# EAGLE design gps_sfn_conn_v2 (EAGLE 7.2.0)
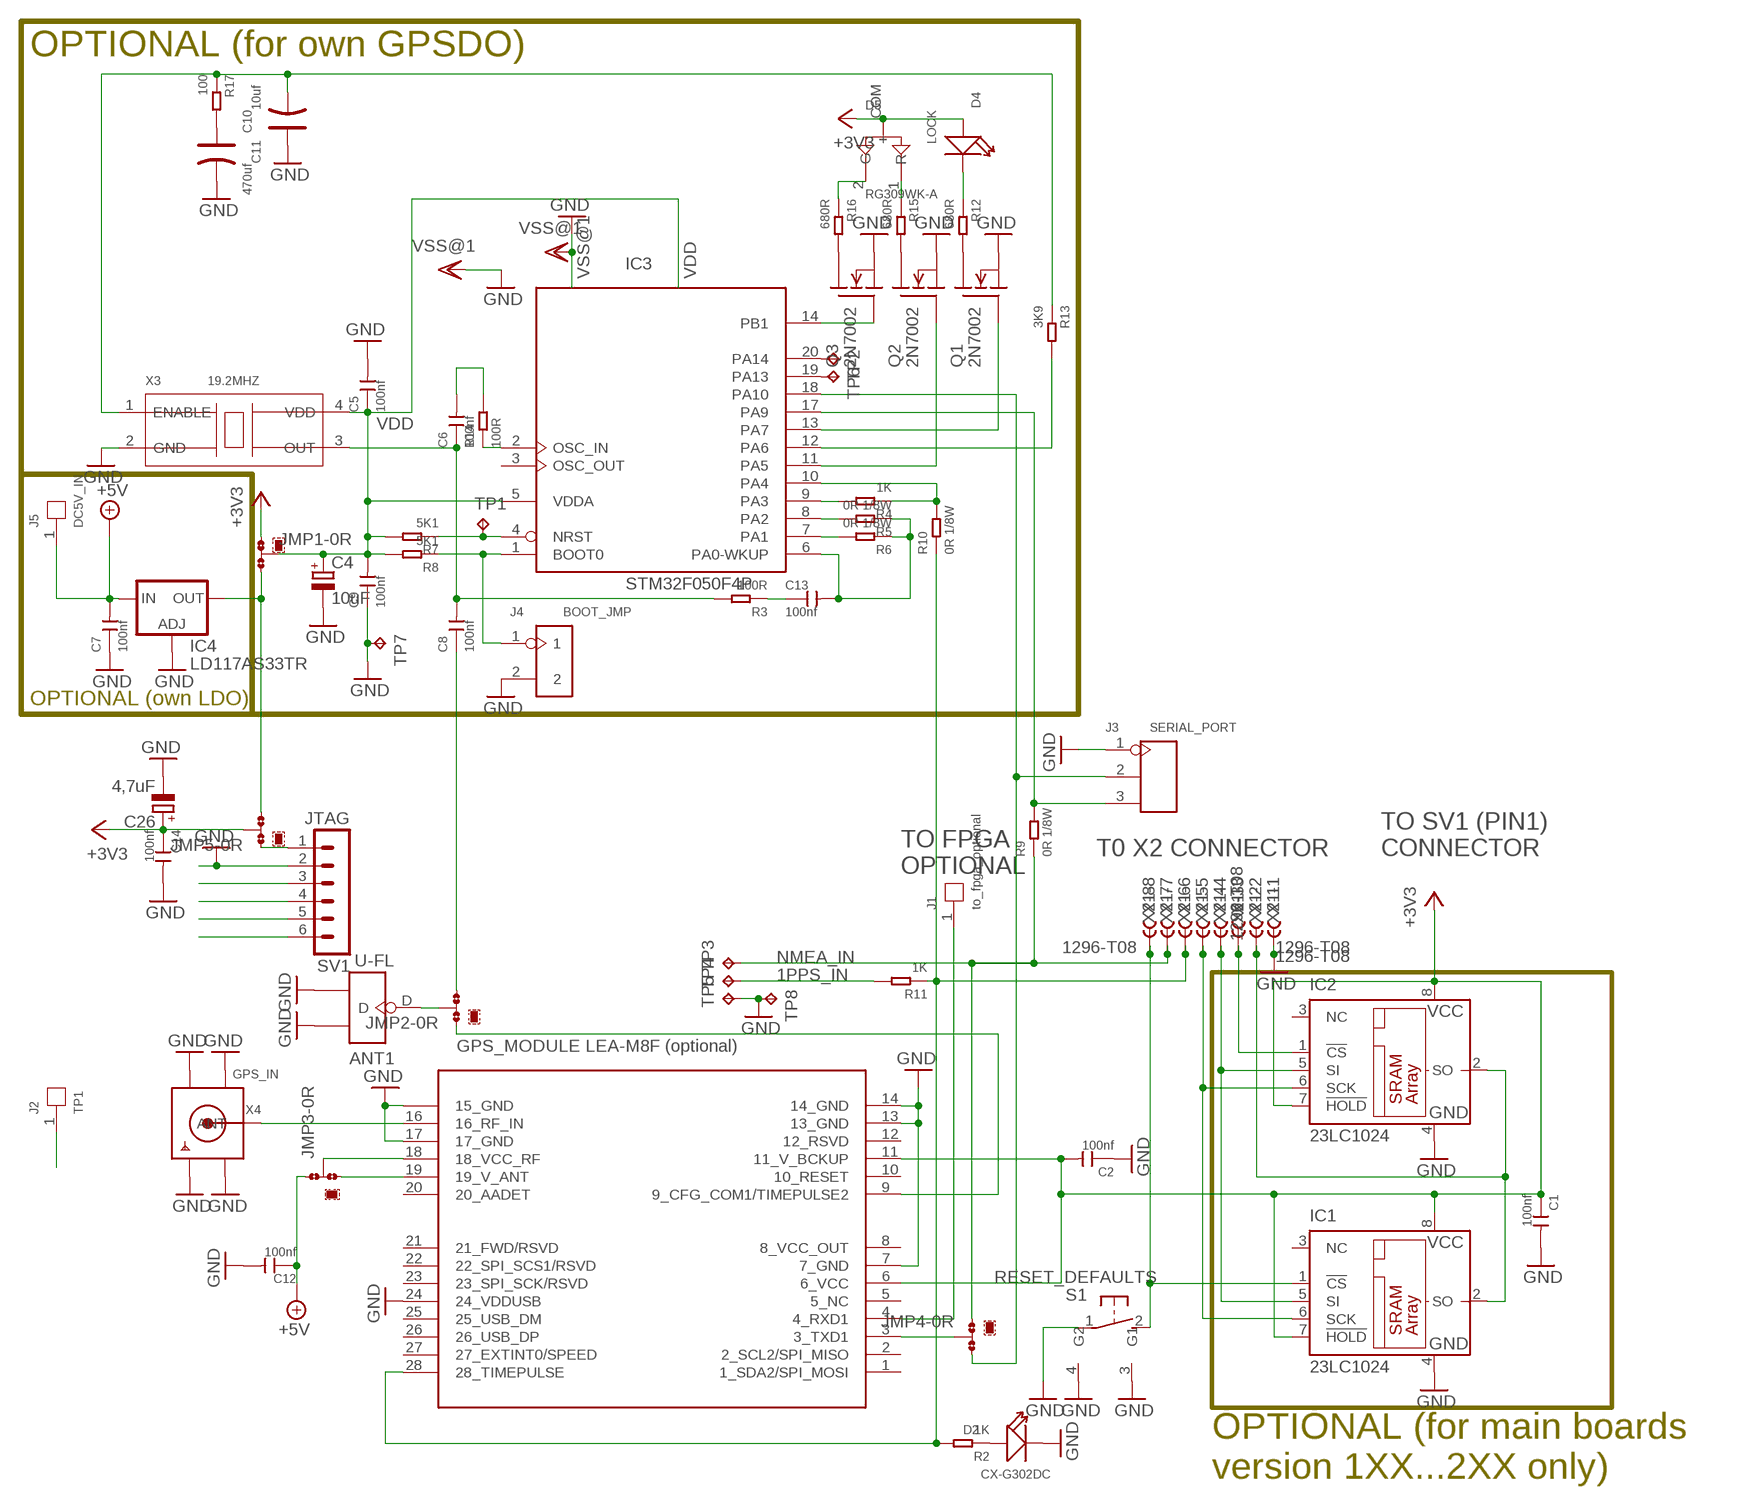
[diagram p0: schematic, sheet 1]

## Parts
ANT1  U-FL  ANTENNA-CONN-U-FL(3P)  [U-FL3P-SMD-2.6X2.6X1.0MM]
C1  100nf  CERAMIC-100NF-50V-10%-X7R(0805)  [C0805]
C2  100nf  CERAMIC-100NF-50V-10%-X7R(0805)  [C0805]
C4  10uF  CPOL-EUA/3216-18R  [A/3216-18R]
C5  100nf  CERAMIC-100NF-50V-10%-X7R(0805)  [C0805]
C6  100nf  CERAMIC-100NF-50V-10%-X7R(0805)  [C0805]
C7  100nf  CERAMIC-100NF-50V-10%-X7R(0805)  [C0805]
C8  100nf  CERAMIC-100NF-50V-10%-X7R(0805)  [C0805]
C9  100nf  CERAMIC-100NF-50V-10%-X7R(0805)  [C0805]
C10  470uf  TANTALUM-SMD-470UF-6.3V(AVX-D)  [AVX-D]
C11  10uf  TANTALUM-SMD-10UF-10V-10%(AVX-A)  [AVX-A]
C12  100nf  CERAMIC-100NF-50V-10%-X7R(0805)  [C0805]
C13  100nf  CERAMIC-100NF-50V-10%-X7R(0805)  [C0805]
C14  100nf  CERAMIC-100NF-50V-10%-X7R(0805)  [C0805]
C26  4,7uF  CPOL-EUA/3216-18R  [A/3216-18R]
D2  CX-G302DC  DIP-LED-GREEN-GREEN(2P-D3MM)  [LED2-2.54-D3.0MM]
D4  LOCK  DIP-LED-GREEN-GREEN(2P-D3MM)  [LED2-2.54-D3.0MM]
D5  RG309WK-A  DIP-LED-RED/GREEN-COMMON-CATHODE(3P-2.54)  [LED3-2.54-D3.0MM]
IC1  23LC1024  23SOIC  [SO-08]
IC2  23LC1024  23SOIC  [SO-08]
IC3  STM32F050F4P  [TSSOP20-I]
IC4  LD117AS33TR  [SOT223]
J1  to_fpga_optional  DIP-BLACK-ROUND-FEMALE-HEADER-VERT(1P-2.54)  [1P-65/35MIL]
J2  TP1  DIP-BLACK-ROUND-FEMALE-HEADER-VERT(1P-2.54)  [1P-65/35MIL]
J3  SERIAL_PORT  DIP-BLACK-FEMALE-HEADER-VERT(3P-2.54)  [H3-2.54]
J4  BOOT_JMP  DIP-BLACK-FEMALE-HEADER-VERT(2P-2.54)  [H2-2.54]
J5  DC5V_IN  DIP-BLACK-ROUND-FEMALE-HEADER-VERT(1P-2.54)  [1P-65/35MIL]
JMP1  0R-JUMPA  [A0R-JMP]
JMP2  0R-JUMPA  [A0R-JMP]
JMP3  0R-JUMPA  [A0R-JMP]
JMP4  0R-JUMPA  [A0R-JMP]
JMP5  0R-JUMPA  [A0R-JMP]
Q1  2N7002  [SOT23]
Q2  2N7002  [SOT23]
Q3  2N7002  [SOT23]
R2  1K  SMD-RES-0R-5%-1/8W(0805)  [R0805]
R3  100R  SMD-RES-0R-5%-1/8W(0805)  [R0805]
R4  1K  SMD-RES-0R-5%-1/8W(0805)  [R0805]
R5  0R 1/8W  SMD-RES-0R-5%-1/8W(0805)  [R0805]
R6  0R 1/8W  SMD-RES-0R-5%-1/8W(0805)  [R0805]
R7  5K1  SMD-RES-0R-5%-1/8W(0805)  [R0805]
R8  5K1  SMD-RES-0R-5%-1/8W(0805)  [R0805]
R9  0R 1/8W  SMD-RES-0R-5%-1/8W(0805)  [R0805]
R10  0R 1/8W  SMD-RES-0R-5%-1/8W(0805)  [R0805]
R11  1K  SMD-RES-0R-5%-1/8W(0805)  [R0805]
R12  680R  SMD-RES-0R-5%-1/8W(0805)  [R0805]
R13  3K9  SMD-RES-0R-5%-1/8W(0805)  [R0805]
R14  100R  SMD-RES-0R-5%-1/8W(0805)  [R0805]
R15  680R  SMD-RES-0R-5%-1/8W(0805)  [R0805]
R16  680R  SMD-RES-0R-5%-1/8W(0805)  [R0805]
R17  100  SMD-RES-0R-5%-1/8W(0805)  [R0805]
S1  RESET_DEFAULTS  31-XX  [B3F-31XX]
SV1  JTAG  MA06-1  [MA06-1]
TP1  UART_OUT  TPB1,27  [B1,27]
TP2  UART_OUT  TPB1,27  [B1,27]
TP3  UART_OUT  TPB1,27  [B1,27]
TP4  UART_OUT  TPB1,27  [B1,27]
TP5  UART_OUT  TPB1,27  [B1,27]
TP6  UART_OUT  TPB1,27  [B1,27]
TP7  UART_OUT  TPB1,27  [B1,27]
TP8  UART_OUT  TPB1,27  [B1,27]
UBLOX_LEA-M8F  UBLOX_LEA-M8F/Quectel L10  UBLOX_LEA-6  [UBLOX_LEA-6T]
X1  1296-T08  [1296-08]
X2  1296-T08  [1296-08]
X3  19.2MHZ  SMD-CRYSTAL-16MHZ-9PF-10PPM-60R(4P-3.2X2.5MM)  [X4-SMD-3.2X2.5X0.7MM]
X4  GPS_IN  SMACONNECTOR_EDGE_UFL  [SMA_EDGELAUNCH_UFL]

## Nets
1PPS_IN: R2.2 R10.1 R11.1 UBLOX_LEA-M8F.28(28_TIMEPULSE) X1.6 X2.6
+3V3: C1.1 C2.2 C14.1 C26.+ D4.A(+) D5.COM(+) IC1.7(!HOLD) IC1.8(VCC) IC2.7(!HOLD) IC2.8(VCC) JMP1.1 JMP5.2 UBLOX_LEA-M8F.6(6_VCC) UBLOX_LEA-M8F.11(11_V_BCKUP)
+5V: C7.2 C12.1 IC4.3(IN) J5.1 JMP3.1
GND: ANT1.GND1 ANT1.GND2 C1.2 C2.1 C4.- C5.2 C7.1 C9.1 C10.- C11.+ C12.2 C14.2 C26.- D2.K(-) IC1.4(GND) IC2.4(GND) IC4.1(ADJ) J3.1 J4.2 Q1.2(S) Q2.2(S) Q3.2(S) S1.1(P) S1.3(G1) S1.4(G2) SV1.2 TP5.TP TP7.TP TP8.TP UBLOX_LEA-M8F.7(7_GND) UBLOX_LEA-M8F.13(13_GND) UBLOX_LEA-M8F.14(14_GND) UBLOX_LEA-M8F.15(15_GND) UBLOX_LEA-M8F.17(17_GND) UBLOX_LEA-M8F.24(24_VDDUSB) X1.1 X2.1 X3.2(GND) X4.GND@1(GND1) X4.GND@2(GND2) X4.GND@3(GND3) X4.GND@4(GND4)
N$1: SV1.6
N$2: SV1.5
N$3: SV1.4
N$4: SV1.3
N$5: IC1.1(!CS) S1.2(S) X1.8 X2.8
N$6: JMP3.3 UBLOX_LEA-M8F.19(19_V_ANT)
N$7: IC1.2(SO) IC2.2(SO) X1.2 X2.2
N$8: IC2.1(!CS) X1.3 X2.3
N$9: IC1.5(SI) IC2.5(SI) X1.4 X2.4
N$10: IC1.6(SCK) IC2.6(SCK) X1.5 X2.5
N$11: J1.1 UBLOX_LEA-M8F.4(4_RXD1)
N$12: D2.A(+) R2.1
N$13: UBLOX_LEA-M8F.16(16_RF_IN) X4.P(ANT)
N$14: JMP3.2 UBLOX_LEA-M8F.18(18_VCC_RF)
N$15: JMP2.1 UBLOX_LEA-M8F.9(9_CFG_COM1/TIMEPULSE2)
N$16: R11.2 TP4.TP
N$17: IC3.20(PA14) TP2.TP
N$18: ANT1.D JMP2.2
N$19: J2.1
N$20: IC3.4(NRST) R7.1 TP1.TP
N$21: IC3.1(BOOT0) J4.1 R8.1
N$22: C13.2 IC3.6(PA0-WKUP) R5.1 R6.1
N$23: JMP4.2 UBLOX_LEA-M8F.3(3_TXD1)
N$24: C13.1 R3.1
N$25: C6.1 C8.2 R3.2 X3.3(OUT)
N$26: IC3.9(PA3) R4.2
N$27: IC3.10(PA4) R4.1 R10.2
N$28: IC3.7(PA1) R6.2
N$29: IC3.2(OSC_IN) R14.1
N$30: IC3.8(PA2) R5.2
N$31: IC4.4(OUT) JMP1.3 JMP5.3
N$32: C6.2 R14.2
N$33: JMP5.1 SV1.1
N$34: C8.1 JMP2.3
N$35: IC3.18(PA10) J3.2 JMP4.3
N$36: IC3.17(PA9) J3.3 R9.2
N$37: IC3.12(PA6) R13.2
N$38: C10.+ R17.2
N$39: C11.- R13.1 R17.1 X3.1(ENABLE)
N$40: D5.1(R) R15.1
N$41: D5.2(G) R16.1
N$42: D4.K(-) R12.1
N$43: IC3.14(PB1) Q3.1(G)
N$44: IC3.11(PA5) Q2.1(G)
N$45: IC3.13(PA7) Q1.1(G)
N$46: IC3.19(PA13) TP6.TP
N$47: Q1.3(D) R12.2
N$48: Q2.3(D) R15.2
N$49: Q3.3(D) R16.2
NMEA_IN: JMP4.1 R9.1 TP3.TP X1.7 X2.7
VDD: C4.+ C5.1 C9.2 IC3.5(VDDA) JMP1.2 R7.2 R8.2 X3.4(VDD)
Unconnected: IC1.3(NC) IC2.3(NC) IC3.3(OSC_OUT) UBLOX_LEA-M8F.1(1_SDA2/SPI_MOSI) UBLOX_LEA-M8F.2(2_SCL2/SPI_MISO) UBLOX_LEA-M8F.5(5_NC) UBLOX_LEA-M8F.8(8_VCC_OUT) UBLOX_LEA-M8F.10(10_RESET) UBLOX_LEA-M8F.12(12_RSVD) UBLOX_LEA-M8F.20(20_AADET) UBLOX_LEA-M8F.21(21_FWD/RSVD) UBLOX_LEA-M8F.22(22_SPI_SCS1/RSVD) UBLOX_LEA-M8F.23(23_SPI_SCK/RSVD) UBLOX_LEA-M8F.25(25_USB_DM) UBLOX_LEA-M8F.26(26_USB_DP) UBLOX_LEA-M8F.27(27_EXTINT0/SPEED)

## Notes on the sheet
- OPTIONAL (for own GPSDO)
- OPTIONAL (own LDO)
- T0 X2 CONNECTOR
- TO SV1 (PIN1)
  CONNECTOR
- TO FPGA
  OPTIONAL
- GPS_MODULE LEA-M8F (optional)
- OPTIONAL (for main boards
  version 1XX...2XX only)

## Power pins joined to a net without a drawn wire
VDD: IC3.16(VDD)
VSS@1: IC3.15(VSS)

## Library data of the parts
ANT1 = Seeed-OPL-Connector:ANTENNA-CONN-U-FL(3P): 320110048
C1 C2 C5-C9 C12-C14 = Seeed-OPL-Capacitor:CERAMIC-100NF-50V-10%-X7R(0805): 302010165; MPN: CC0805KRX7R9BB104
C4 C26 = rcl:CPOL-EU: POLARIZED CAPACITOR, European symbol
C10 = Seeed-OPL-Capacitor:TANTALUM-SMD-470UF-6.3V(AVX-D): 302020027
C11 = Seeed-OPL-Capacitor:TANTALUM-SMD-10UF-10V-10%(AVX-A): 302020011; MPN: TAJA106K010RNJ
D2 = Seeed-OPL-Diode:DIP-LED-GREEN-GREEN(2P-D3MM): 304090040; MPN: CX-G302DC
D4 = Seeed-OPL-Diode:DIP-LED-GREEN-GREEN(2P-D3MM): 304090040; MPN: CX-G302DC; VALUE: CX-G302DC
D5 = Seeed-OPL-Diode:DIP-LED-RED/GREEN-COMMON-CATHODE(3P-2.54): 304090022; MPN: RG309WK-A
IC1 IC2 = W5500_LX9_AD9957:23*: Serial EEPROM 4K/ 8K , SPI bus
IC3 = micro-stm_v3:STM32F050F*P: ARM 32-bit Cortex™-M0 CPU 48 MHz maximum frequency 16to 32 Kbytes of Flash memory 4 kbytes of SRAM 15 GPIOs 2.0 to 3.6 V application supply
IC4 = W5500_LX9_AD9957:LD117A?*: Low drop fixed and adjustable positive voltage regulators 1 A Source: http://www.st.com/stonline/products/literature/ds/7194/ld1117axx.pdf
J1 J2 J5 = Seeed-OPL-Connector:DIP-BLACK-ROUND-FEMALE-HEADER-VERT(1P-2.54): 320030026; MPN: RF130-1013BBS0741; VALUE: 1p-2.54
J3 = Seeed-OPL-Connector:DIP-BLACK-FEMALE-HEADER-VERT(3P-2.54): 320030024; MPN: F185-1103A0BSYA1; VALUE: 3p-2.54
J4 = Seeed-OPL-Connector:DIP-BLACK-FEMALE-HEADER-VERT(2P-2.54): 320030023; MPN: F185-1102A1BSYA1; VALUE: 2p-2.54
JMP1-JMP5 = W5500_LX9_AD9957:0R-JUMP: SMD 0R 0805 Jumper
Q1-Q3 = transistors_gaui:2N7002
R2-R4 R7 R8 R11-R17 = Seeed-OPL-Resistor:SMD-RES-0R-5%-1/8W(0805): 301010359; MPN: RC0805JR-070RL; VALUE: 0R 1/8W
R5 R6 R9 R10 = Seeed-OPL-Resistor:SMD-RES-0R-5%-1/8W(0805): 301010359; MPN: RC0805JR-070RL
S1 = W5500_LX9_AD9957:31-XX: OMRON SWITCH Now with beefier pads!
SV1 = con-lstb:MA06-1: PIN HEADER; OC_FARNELL: unknown; OC_NEWARK: unknown
TP1-TP8 = testpad:TP: Test pad
UBLOX_LEA-M8F = Ava:UBLOX_LEA-6
X1 X2 = W5500_LX9_AD9957:1296-T08: 1.27mm SINGLE ROW FEMALE SOCKET Source: http://www.leotronics.co.uk/Conexcon/Data%20Sheets/sec.%20A/1296ing.pdf; OC_FARNELL: unknown; OC_NEWARK: unknown
X3 = Seeed-OPL-crystal-osctllator:SMD-CRYSTAL-16MHZ-9PF-10PPM-60R(4P-3.2X2.5MM): 306010078; VALUE: 16MHZ
X4 = W5500_LX9_AD9957:SMACONNECTOR: SMA Connector 90° DIP SMA Connector, 50 Ohm (4UConnector: 07259)

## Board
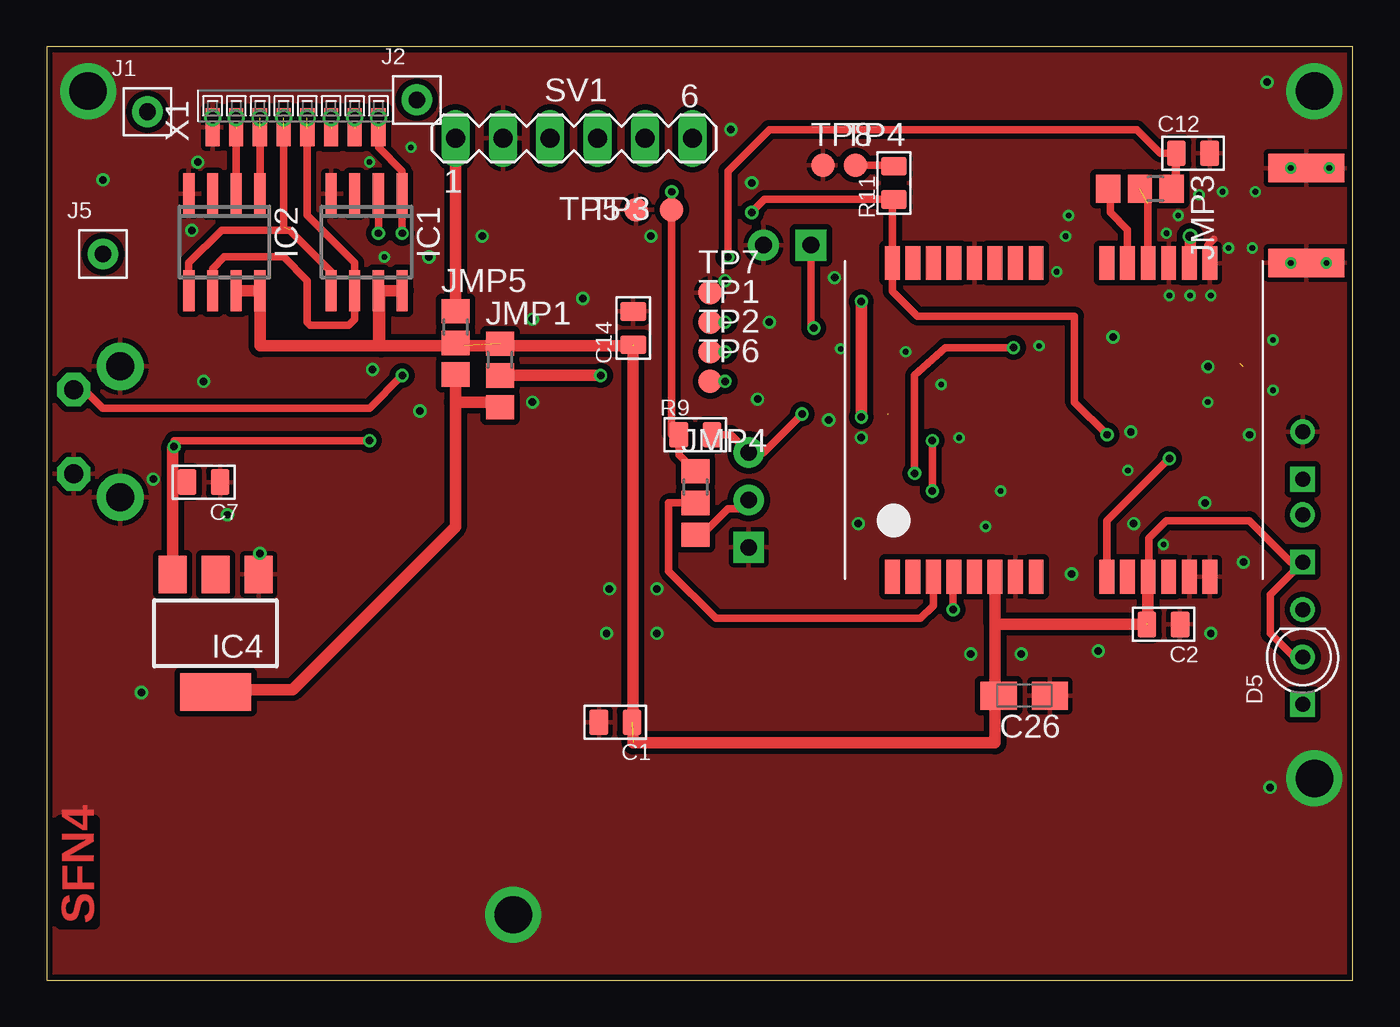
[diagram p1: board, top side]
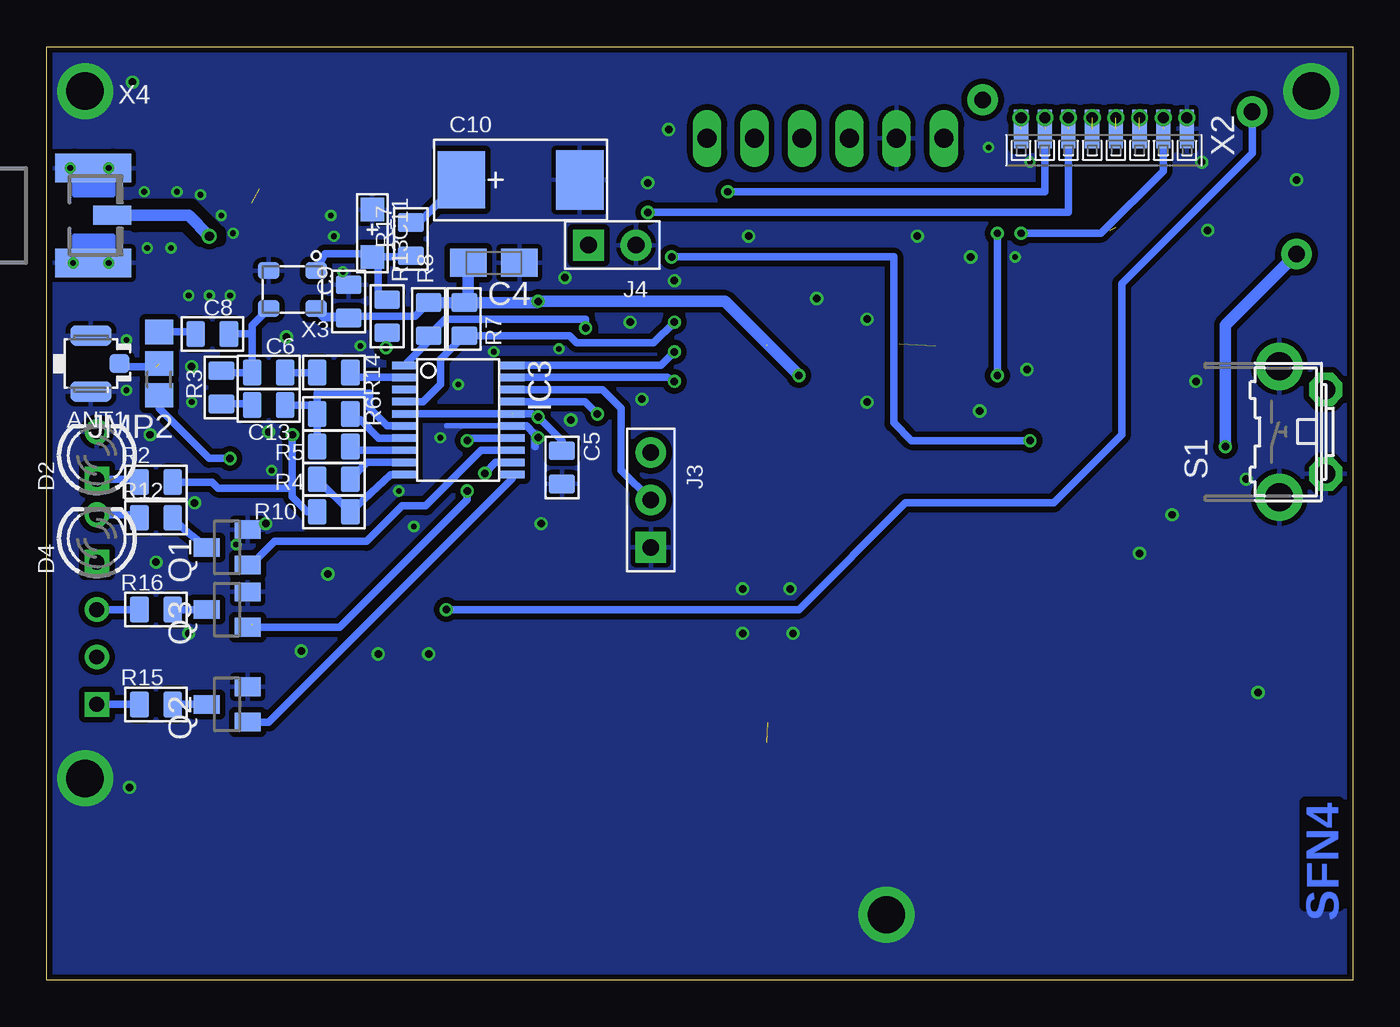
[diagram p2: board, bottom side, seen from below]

Size 70 x 50 mm. Coordinates in mm from the lower left corner, seen from the top.
Outline: 0,0 70,0 70,50 0,50 0,0
Copper layers (1*16): Top 0.035mm / dielectric 1.5mm / Bottom 0.035mm
Design rules "SeeedStudio_2layer_DRU_no_angle_20140221": minimum track width 6mil, minimum drill 12mil, track to track 6mil, track to pad 6mil, pad to pad 6mil, via to via 6mil, smd to smd 0mil, copper to edge 10mil, drill to drill 10mil, minimum pad ring 10mil, minimum via ring 6mil, stop-mask expansion 2mil, vias tented up to drill 100mil, thermal gap 10mil
bRestrict: 5 lines

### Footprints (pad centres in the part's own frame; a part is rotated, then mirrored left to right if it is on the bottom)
U-FL3P-SMD-2.6X2.6X1.0MM = smd 1.05 x 1: D -1.524,0 | smd 2.2 x 1.05: GND1 0,1.5; GND2 0,-1.5
C0805 = smd 1.397 x 1.016: 1 0,0.889; 2 0,-0.889
A/3216-18R = smd 1.95 x 1.5: + 1.375,0; - -1.375,0
AVX-D = smd 2.54 x 3.048: + -3.175,0 | smd 2.54 x 3.175: - 3.175,0
AVX-A = smd 1.27 x 1.27: + -1.27,0; - 1.27,0
LED2-2.54-D3.0MM = drill 0.813 square: A -1.27,0 | drill 0.813: K 1.27,0
LED3-2.54-D3.0MM = drill 0.8 pad 1.3 square: 1 -2.54,0 | drill 0.8 pad 1.3: 2 2.54,0; COM 0,0
SO-08 = smd 0.6 x 2.2: 1 -1.905,-2.6; 2 -0.635,-2.6; 3 0.635,-2.6; 4 1.905,-2.6; 5 1.905,2.6; 6 0.635,2.6; 7 -0.635,2.6; 8 -1.905,2.6
TSSOP20-I = smd 0.4 x 1.35: 1 -2.925,-2.875; 2 -2.275,-2.875; 3 -1.625,-2.875; 4 -0.975,-2.875; 5 -0.325,-2.875; 6 0.325,-2.875; 7 0.975,-2.875; 8 1.625,-2.875; 9 2.275,-2.875; 10 2.925,-2.875; 11 2.925,2.875; 12 2.275,2.875; 13 1.625,2.875; 14 0.975,2.875; 15 0.325,2.875; 16 -0.325,2.875; 17 -0.975,2.875; 18 -1.625,2.875; 19 -2.275,2.875; 20 -2.925,2.875
SOT223 = smd 1.5 x 2: 1 -2.3,-3.15; 2 0,-3.15; 3 2.3,-3.15 | smd 3.8 x 2: 4 0,3.15
1P-65/35MIL = drill 0.889 pad 1.651: 1 0,0
H3-2.54 = drill 0.889 pad 1.651 square: 1 0,2.54 | drill 0.889 pad 1.651: 2 0,0; 3 0,-2.54
H2-2.54 = drill 0.889 pad 1.651 square: 1 0,1.27 | drill 0.889 pad 1.651: 2 0,-1.27
A0R-JMP = smd 1.5 x 1.3: 1 0,1.7; 2 0,0; 3 0,-1.7
SOT23 = smd 1 x 1.4: 1 -0.95,-1.1; 2 0.95,-1.1; 3 0,1.1
R0805 = smd 1.397 x 1.016: 1 0,0.889; 2 0,-0.889
B3F-31XX = drill 1.016 pad 1.778 octagon: 1 -2.261,-1.245; 2 2.261,-1.245 | drill 1.499 pad 2.54: 3 -3.505,1.245; 4 3.505,1.245
MA06-1 = drill 1.016 long: 1 -6.35,0; 2 -3.81,0; 3 -1.27,0; 4 1.27,0; 5 3.81,0; 6 6.35,0
B1,27 = smd 1.27 x 1.27: TP 0,0
UBLOX_LEA-6T = smd 1.8 x 0.8: 1 8.4,-8.65; 2 8.4,-7.55; 3 8.4,-6.45; 4 8.4,-5.35; 5 8.4,-4.25; 6 8.4,-3.15; 7 8.4,-2.05; 8 8.4,-0.95; 9 8.4,2.85; 10 8.4,3.95; 11 8.4,5.05; 12 8.4,6.15; 13 8.4,7.25; 14 8.4,8.35; 15 -8.4,8.35; 16 -8.4,7.25; 17 -8.4,6.15; 18 -8.4,5.05; 19 -8.4,3.95; 20 -8.4,2.85; 21 -8.4,-0.95; 22 -8.4,-2.05; 23 -8.4,-3.15; 24 -8.4,-4.25; 25 -8.4,-5.35; 26 -8.4,-6.45; 27 -8.4,-7.55; 28 -8.4,-8.65
1296-08 = smd 0.76 x 2.05: 1 -1.905,-1.78; 2 -0.635,-1.78; 3 0.635,-1.78; 4 1.905,-1.78; 5 3.175,-1.78; 6 4.445,-1.78; 7 5.715,-1.78; 8 6.985,-1.78
X4-SMD-3.2X2.5X0.7MM = smd 1.143 x 0.889: 1 -1.27,-1.016; 2 1.27,-1.016; 3 1.27,1.016; 4 -1.27,1.016
SMA_EDGELAUNCH_UFL = smd 4.064 x 1.524: GND@1 2.032,-2.54; GND@2 2.032,2.54 | smd 4.064 x 1.524 bottom: GND@3 2.032,2.54; GND@4 2.032,-2.54 | smd 2.032 x 1.016: P 3.048,0

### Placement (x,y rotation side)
ANT1  67.63,33.02 180 bottom
C1  30.48,13.81 270 top
C2  59.85,19.05 270 top
C4  46.04,38.42 180 bottom
C5  42.39,27.46 0 bottom
C6  58.1,32.54 90 bottom
C7  8.41,26.67 270 top
C8  61.12,34.61 90 bottom
C9  53.82,36.35 0 bottom
C10  44.61,42.86 0 bottom
C11  52.55,40.01 270 bottom
C12  61.44,44.29 90 top
C13  58.1,30.8 90 bottom
C14  31.43,34.92 180 top
C26  52.39,15.24 180 top
D2  67.31,28.1 90 bottom
D4  67.31,23.65 90 bottom
D5  67.31,17.3 90 top
IC1  17.14,39.53 180 top
IC2  9.53,39.53 180 top
IC3  47.94,30 270 bottom
IC4  9.05,18.57 180 top
J1  5.4,46.51 0 top
J2  19.84,47.15 0 top
J3  37.62,25.72 180 bottom
J4  39.69,39.37 90 bottom
J5  3.02,38.89 0 top
JMP1  24.29,32.38 0 top
JMP2  63.98,33.02 180 bottom
JMP3  58.58,42.39 270 top
JMP4  34.77,25.56 0 top
JMP5  21.91,34.13 0 top
Q1  60.33,23.18 90 bottom
Q2  60.33,14.76 90 bottom
Q3  60.33,19.84 90 bottom
R2  64.14,26.67 90 bottom
R3  60.64,31.75 180 bottom
R4  54.61,26.83 90 bottom
R5  54.61,28.57 90 bottom
R6  54.61,30.32 90 bottom
R7  47.62,35.4 180 bottom
R8  49.53,35.4 180 bottom
R9  34.77,29.21 90 top
R10  54.61,25.08 90 bottom
R11  45.4,42.7 180 top
R12  64.14,24.77 90 bottom
R13  51.75,35.56 0 bottom
R14  54.61,32.54 270 bottom
R15  64.14,14.76 90 bottom
R16  64.14,19.84 90 bottom
R17  50.48,39.69 180 bottom
S1  2.7,29.37 90 bottom
SV1  28.26,45.09 0 top
TP1  35.56,35.24 0 top
TP2  35.56,33.66 0 top
TP3  33.5,41.27 0 top
TP4  43.34,43.66 0 top
TP5  31.59,41.27 0 top
TP6  35.56,32.07 0 top
TP7  35.56,36.83 0 top
TP8  41.59,43.66 0 top
UBLOX_LEA-M8F  53.98,30 270 top
X1  10.79,47.47 0 top
X2  10.79,43.81 180 bottom
X3  56.83,36.99 180 bottom
X4  69.53,40.96 0 bottom

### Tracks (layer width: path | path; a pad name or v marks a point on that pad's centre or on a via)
1PPS_IN  (via drill 0.4, 0.6)  (1 unrouted)
  Top 0.406: X1.6 v15.24,46.2 | 45.4,38.4 UBLOX_LEA-M8F.28 | 45.33,42.07 45.33,41.75 | 45.33,41.75 45.4,41.75 R11.1 | R11.1 45.4,41.91 | v56.83,29.21 55.09,30.96 55.09,35.56 46.67,35.56 45.33,36.91 UBLOX_LEA-M8F.28 | v37.78,41.12 38.48,41.81 R11.1 | 45.33,41.75 UBLOX_LEA-M8F.28
  Bottom 0.406: v15.24,46.2 15.24,41.12 v37.78,41.12 | R2.2 61.12,26.67 60.8,26.35 56.83,26.35 | 56.83,26.35 v56.83,29.21 | R10.1 56.04,25.08 56.83,25.88 56.83,26.35
+3V3  (4 unrouted)
  Top 0.406: UBLOX_LEA-M8F.11 59.05,21.63 59.05,23.65 60.01,24.61 64.45,24.61 66.67,22.38 D4.A 65.56,20.64 65.56,18.57 66.83,17.3 D5.COM | JMP5.2 22.07,33.97 22.38,33.97 | IC1.8 18.99,36.99 17.78,36.99 17.94,36.83 17.94,33.97 | C26.+ 51.01,14.95 50.83,14.76
  Top 0.61: IC1.8 IC1.7 17.78,34.13 | 11.43,35.4 IC2.8 | IC2.8 IC2.7 | UBLOX_LEA-M8F.11 59.02,19.05 50.83,19.05 | 50.83,19.05 UBLOX_LEA-M8F.6 | IC2.8 11.43,33.97 17.94,33.97 22.38,33.97 31.43,33.97 31.43,12.7 50.83,12.7 50.83,14.76 50.83,19.05
+5V  (via drill 0.4)
  Top 0.406: C12.1 60.55,42.66 JMP3.1 60.48,42.59 60.48,44.29 59.69,44.29 58.42,45.56 38.73,45.56 36.51,43.34 v36.51,38.73 | v17.3,28.89 6.83,28.89 v6.83,28.57 6.83,28.42 | C7.2 7.37,26.83 6.75,26.83
  Top 0.61: IC4.3 6.75,26.83 6.75,28.5 v6.83,28.57
  Bottom 0.406: v17.3,28.89 23.65,28.89 24.61,29.84 24.61,38.73 v36.51,38.73
  Bottom 0.61: J5.1 6.83,35.08 v6.83,28.57
GND  (via drill 0.3, 0.4, 0.6, 2)
  Top 0.406: 62.55,39.69 62.23,39.37 62.23,39.05
  Top 0.61: UBLOX_LEA-M8F.24 49.69,38.37
  Bottom 0.305: 44.29,29.69 48.58,29.69
  Bottom 0.406: 44.29,29.69 43.81,29.21 43.81,28.57
  other vias: 65.41,48.1 3.02,42.86 9.68,24.92 5.71,26.83 11.43,22.86 67.94,47.62 67.94,10.79 2.22,47.62 65.56,10.32 5.08,15.4 8.89,46.2 17.46,32.7 18.1,38.73 17.3,43.81 8.1,43.81 7.78,40.16 57.15,34.45 62.23,32.86 64.45,29.21 8.41,32.07 20,30.48 20.48,38.73 23.34,39.85 26.04,30.96 26.04,35.4 32.38,39.85 28.73,36.51 37.78,42.7 36.35,37.47 36.67,45.56 58.26,24.45 54.93,21.75 62.07,25.56 52.23,17.46 56.36,17.62 64.14,22.38 43.66,29.05 43.5,24.45 32.7,20.95 32.7,18.57 42.23,37.62 38.73,35.24 38.1,31.11 41.91,30 62.39,18.57 64.77,42.23 25,3.5 58.1,29.37 63.02,42.23 61.75,42.07 60.64,40.96 60.01,40.01 60.17,36.67 61.28,36.67 62.39,36.67 63.34,39.21 64.61,39.21 66.67,38.42 68.58,38.42 68.74,43.5 66.67,43.5 53.18,33.97 46.04,33.66 42.55,33.81 48.9,29.05 47.94,31.91 51.12,26.19 50.32,24.29 19.53,44.61 30,18.57 30.16,20.95 49.53,17.46 65.72,34.29 65.72,31.59 62.23,30.96 57.94,27.3 54.77,40.96 54.61,39.85 59.85,23.34 54.13,37.94
  pour Top (isolate 0.305): 0,50 70,50 70,0 0,0
  pour Bottom (isolate 0.305): 0,50 70,50 70,0 0,0
N$5  (via drill 0.4, 0.6)  (1 unrouted)
  Top 0.406: v17.78,46.2 17.78,44.61 19.05,43.34 IC1.1 v19.05,40.01 | v19.05,32.38 17.3,30.64 3.02,30.64 2.03,31.63 S1.2
  Bottom 0.406: v17.78,46.2 17.75,46.23 X2.8 | v19.05,40.01 v19.05,32.38
N$6
  Top 0.406: UBLOX_LEA-M8F.19 57.92,40.18 56.99,41.12 56.99,41.86 JMP3.3
N$7  (via drill 0.4, 0.6)  (1 unrouted)
  Top 0.406: X1.2 v10.16,46.2 IC2.2 | IC1.2 v17.78,40.01
  Bottom 0.406: v17.78,40.01 13.49,40.01 10.16,43.34 v10.16,46.2
N$8  (via drill 0.6)  (2 unrouted)
  Top 0.406: X1.3 IC2.1
  other vias: 11.43,46.2
N$9  (via drill 0.6)  (3 unrouted)
  Top 0.406: X1.4 12.7,40.32 | IC1.5 15.24,37.94 13.02,40.16 9.37,40.16 7.62,38.42 IC2.5
  other vias: 12.7,46.2
N$10  (via drill 0.6)  (2 unrouted)
  Top 0.406: X1.5 13.97,40.96 16.51,38.42 IC1.6 16.51,35.4 16.19,35.08 14.13,35.08 13.97,35.24 13.97,37.47 12.7,38.73 9.53,38.73 8.89,38.1 IC2.6
  other vias: 13.97,46.2
N$11  (via drill 0.4)
  Top 0.406: UBLOX_LEA-M8F.4 48.58,21.6 v48.58,19.84
  Bottom 0.406: J1.1 5.4,44.29 12.38,37.31 12.38,29.21 16.03,25.56 23.97,25.56 29.69,19.84 v48.58,19.84
N$12
  Bottom 0.406: D2.A 65.18,26.83 R2.1
N$13  (via drill 0.5)
  Top 0.61: v61.28,39.85 61.28,38.46 UBLOX_LEA-M8F.16
  Bottom 0.61: X4.P 62.39,40.96 v61.28,39.85
N$14  (1 unrouted)
  Top 0.406: UBLOX_LEA-M8F.18 59.02,41.62
N$15  (via drill 0.4)
  Top 0.406: v60.17,27.94 56.83,24.6 UBLOX_LEA-M8F.9
  Bottom 0.406: 63.5,31.27 63.98,31.27 JMP2.1 63.98,30.64 61.28,27.94 v60.17,27.94
N$16
  Top 0.406: R11.2 45.34,43.66 TP4.TP
N$17  (via drill 0.4)
  Top 0.406: v36.35,33.66 TP2.TP
  Bottom 0.406: IC3.20 37.08,32.93 v36.35,33.66
N$18  (1 unrouted)
  Bottom 0.406: ANT1.D 66.1,32.86 64.14,32.86 | 64.14,32.86 64.14,33.5 | 64.13,32.86 64.14,32.86
N$20  (via drill 0.4)
  Top 0.406: v36.35,35.24 TP1.TP
  Bottom 0.406: IC3.4 49.83,30.98 48.9,31.91 48.9,33.24 R7.1 41.97,34.51 41.59,34.13 37.47,34.13 v36.35,35.24
N$21  (via drill 0.4)
  Top 0.406: v41.12,34.92 40.96,35.08 J4.1
  Bottom 0.406: IC3.1 49.53,34.22 R8.1 48.64,35.4 41.12,35.4 v41.12,34.92
N$22
  Bottom 0.406: 55.5,29.69 R6.1 arc-90 55.98,30.8 C13.2 | 55.5,29.69 R5.1 | 55.5,29.69 55.49,29.68 55.49,31.43 52.7,31.43 52.7,30.64 51.74,29.68 IC3.6
N$23
  Top 0.406: JMP4.2 33.34,25.56 33.34,21.91 35.88,19.37 46.83,19.37 47.52,20.06 UBLOX_LEA-M8F.3
N$24
  Bottom 0.406: R3.1 59.05,30.86 C13.1
N$25
  Bottom 0.406: C8.2 58.99,34.61 | 58.99,34.61 C6.1 60.55,32.54 R3.2 | X3.3 58.99,35.08 58.99,34.61
N$26
  Bottom 0.406: R4.2 52.82,27.73 IC3.9
N$27
  Bottom 0.406: IC3.10 51.57,27.08 R10.2 53.72,25.05 R4.1
N$28
  Bottom 0.406: IC3.7 52.21,29.03 53.18,30 53.4,30 R6.2
N$29
  Bottom 0.406: IC3.2 53.72,32.28 R14.1
N$30
  Bottom 0.406: IC3.8 53.52,28.38 arc90 R5.2
N$31
  Top 0.61: JMP5.3 21.91,30.96 | 21.91,30.96 21.91,24.29 13.18,15.56 9.18,15.56 IC4.4 | JMP1.3 24.02,30.96 21.91,30.96
N$32
  Bottom 0.406: C6.2 R14.2
N$33
  Top 0.61: SV1.1 JMP5.1
N$34
  Bottom 0.406: JMP2.3 62.12,34.72 C8.1
N$35
  Top 0.406: JMP4.3 35.13,23.86 36.51,25.24 37.15,25.24 J3.2
  Bottom 0.406: IC3.18 40.2,31.63 39.21,30.64 39.21,27.3 J3.2
N$36  (via drill 0.4)
  Top 0.406: R9.2 36.67,29.21 J3.3 38.42,28.26 v40.48,30.32
  Bottom 0.406: IC3.17 41.14,30.98 v40.48,30.32
N$37  (via drill 0.4)
  Top 0.406: v51.82,33.88 48.16,33.88 46.51,32.38 v46.51,27.15
  Bottom 0.406: v51.82,33.88 R13.2 | v46.51,27.15 45.93,27.73 IC3.12
N$38
  Bottom 0.406: C10.+ 50.07,40.58 R17.2
N$39
  Bottom 0.406: X3.1 55.09,38.89 52.7,38.89 C11.- | C11.- 50.55,38.73 R17.1 | R13.1 52.23,36.45 52.23,38.42 C11.-
N$40
  Bottom 0.406: D5.1 R15.1
N$41
  Bottom 0.406: D5.2 R16.1
N$42
  Bottom 0.406: D4.K 65.18,24.92 R12.1
N$43  (via drill 0.4)
  Top 0.406: v47.47,26.19 v47.47,28.89
  Bottom 0.406: Q3.1 54.29,18.89 47.47,25.72 v47.47,26.19 | IC3.14 47.33,29.03 v47.47,28.89
N$44
  Bottom 0.406: IC3.11 45.07,26.85 58.1,13.81 Q2.1
N$45
  Bottom 0.406: IC3.13 46.71,28.38 49.69,25.4 50.96,25.4 52.86,23.5 57.78,23.5 58.9,22.38 59.07,22.23 Q1.1
N$46  (via drill 0.4)
  Top 0.406: v36.35,32.07 TP6.TP
  Bottom 0.406: IC3.19 36.72,32.28 v36.35,32.07
N$47
  Bottom 0.406: R12.2 62.54,24.05 Q1.3
N$48
  Bottom 0.406: R15.2 Q2.3
N$49
  Bottom 0.406: R16.2 Q3.3
NMEA_IN  (via drill 0.4, 0.6)  (1 unrouted)
  Top 0.406: X1.7 v16.51,46.2 | v33.5,42.23 TP3.TP 33.5,29.21 R9.1 33.88,28.15 JMP4.1
  Bottom 0.406: v16.51,46.2 16.51,42.23 v33.5,42.23
VDD  (via drill 0.4)  (1 unrouted)
  Top 0.61: 24.35,32.32 JMP1.2 v29.69,32.38 | v43.66,36.35 v43.66,30.16
  Bottom 0.406: IC3.16 43.98,30.33 v43.66,30.16 42.39,28.89 C5.1 | R8.2 50.26,35.56 55.24,35.56 | IC3.16 45.08,30.33 IC3.5 | 55.24,35.56 55.15,35.47 C9.2 | 55.24,35.56 55.56,35.88 X3.4
  Bottom 0.61: v29.69,32.38 33.66,36.35 v43.66,36.35 43.72,36.29 R7.2 | R7.2 47.41,36.5 C4.+ | R7.2 R8.2

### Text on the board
Top: SFN4
Bottom: SFN4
